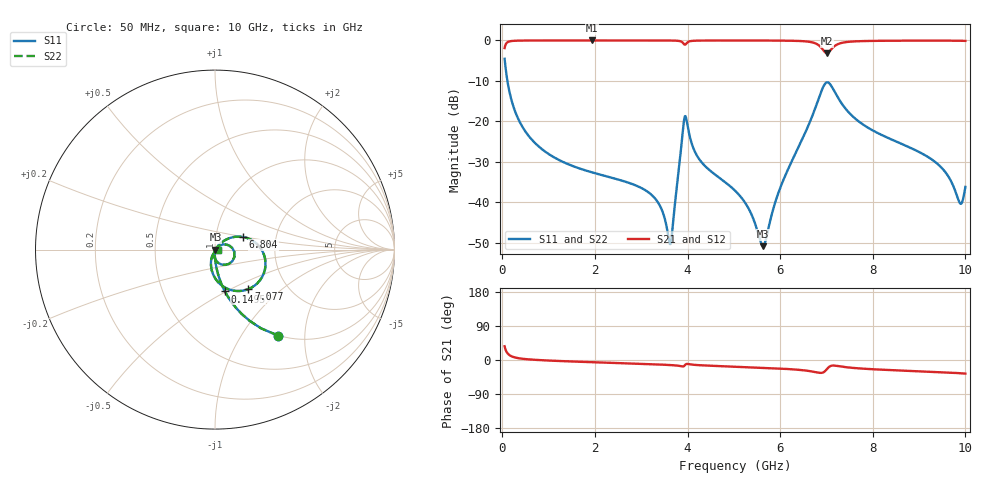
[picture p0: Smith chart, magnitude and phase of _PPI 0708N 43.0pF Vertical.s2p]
! S-Parameter data specifications (vertical orientation):
! Substrate: 40-mil Rogers 3003C, Substrate thickness, H=1.016mm, Dielectric constant, Er=3, Conductor thickness, T_mtl=0.043mm, Loss Tangent, Tand=0.003
! PCB Mounting Pad Footprint: Pad width, PadW=2.54mm , Pad length, PadL=0.51mm , Pad gap, PadG (edge-to-edge)=0.71mm , Reference planes=1.73mm apart
! Created Fri Jan 19 10:18:43 2018
# GHz S MA R 50
! 2 Port Network Data from SP1.SP block
! freq  magS11  angS11  magS21  angS21  magS12  angS12  magS22  angS22
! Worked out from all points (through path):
!   801 points, 50 MHz to 10 GHz, reference 50 ohm
!   highest |S21| = -0.01 dB at 1.928 GHz (marker M1); lowest = -3.1 dB at 7.003 GHz (marker M2)
!   group delay of S21, straight-line fit = 10.3 ps
!   lowest |S11| = -50.8 dB at 5.634 GHz (marker M3), VSWR 1.01, Z = 50.3 - j0.117 ohm
!   |S11| at or under -10 dB: 110.7 MHz to end of sweep
!   |S22| runs from -50.8 to -4.5 dB; largest |S21 - S12| = 0
!   S11 on the Smith chart (normalised r, x): 50 MHz: 1.00, -1.47; 149.5 MHz: 1.00, -0.49; 6.804 GHz: 1.36, +0.20; 7.077 GHz: 1.29, -0.62; 10 GHz: 1.03, -0.00
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0.05  0.5932 -53.8  0.8049 36.2  0.8049 36.2  0.5932 -53.8
0.1495  0.2396 -76.6  0.9707 13.3  0.9707 13.3  0.2396 -76.6
0.647  0.05868 -88.7  0.9979 1.0  0.9979 1.0  0.05868 -88.7
1.716625  0.02565 -93.8  0.9991 -4.9  0.9991 -4.9  0.02565 -93.8
1.928063  0.02354 -94.5  0.9991 -5.8  0.9991 -5.8  0.02354 -94.5
3.370812  0.009794 -94.2  0.9985 -11.9  0.9985 -11.9  0.009794 -94.2
3.632  0.003051 -20.2  0.9968 -13.3  0.9968 -13.3  0.003051 -20.2
3.893187  0.07131 22.6  0.9438 -16.9  0.9438 -16.9  0.07131 22.6
3.955375  0.1162 -33.8  0.8909 -12.1  0.8909 -12.1  0.1162 -33.8
4.253875  0.03403 -96.8  0.9952 -13.7  0.9952 -13.7  0.03403 -96.8
5.025  0.01395 -100.0  0.9978 -17.6  0.9978 -17.6  0.01395 -100.0
5.634437  0.002874 -23.9  0.9969 -20.5  0.9969 -20.5  0.002874 -23.9
6.007562  0.0154 48.2  0.9946 -22.7  0.9946 -22.7  0.0154 48.2
6.691625  0.1158 35.9  0.9474 -30.4  0.9474 -30.4  0.1158 35.9
6.803562  0.172 24.0  0.8954 -32.9  0.8954 -32.9  0.172 24.0
7.002562  0.3025 -26.1  0.6972 -25.0  0.6972 -25.0  0.3025 -26.1
7.077187  0.2884 -49.7  0.7458 -16.5  0.7458 -16.5  0.2884 -49.7
7.375687  0.1526 -91.2  0.9443 -18.2  0.9443 -18.2  0.1526 -91.2
8.345812  0.06186 -110.1  0.9909 -26.4  0.9909 -26.4  0.06186 -110.1
9.415437  0.02926 -112.1  0.9942 -31.9  0.9942 -31.9  0.02926 -112.1
9.888063  0.009674 -58.1  0.9907 -34.9  0.9907 -34.9  0.009674 -58.1
10  0.01552 -3.2  0.9865 -36.0  0.9865 -36.0  0.01552 -3.2
